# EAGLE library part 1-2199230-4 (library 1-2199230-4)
M.2 NGFF, M.2 Connectors, Height 4.2 mm [.165 in], Keying Code M, Gold, Board-to-Board, 67 Position, .02 in [.5 mm] Centerline, Printed Circuit Board Source: Datasheet
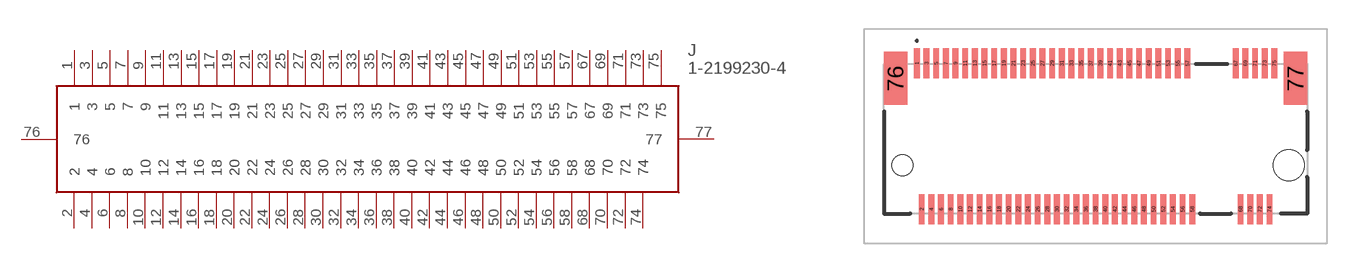
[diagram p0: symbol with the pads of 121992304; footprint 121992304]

Designator prefix J

## 1-2199230-4 (Arrow_Part_Number: 1-2199230-4; Arrow_Price-Stock: https://www.arrow.com/en/products/1-2199230-4/te-connectivity?region=nac; Description: M.2 NGFF, M.2 Connectors, Height 4.2 mm [.165 in], Keying Code M, Gold, Board-to-Board, 67 Position, .02 in [.5 mm] Centerline, Printed Circuit Board; Height: mm; Manufacturer_Name: TE Connectivity; Manufacturer_Part_Number: 1-2199230-4; Mouser_Part_Number: 571-1-2199230-4; Mouser_Price-Stock: https://www.mouser.co.uk/ProductDetail/TE-Connectivity/1-2199230-4?qs=gAfoL%252BRo%2FrJHWNmRjPOT7g%3D%3D)  [121992304]
1  1
2  2
3  3
4  4
5  5
6  6
7  7
8  8
9  9
10  10
11  11
12  12
13  13
14  14
15  15
16  16
17  17
18  18
19  19
20  20
21  21
22  22
23  23
24  24
25  25
26  26
27  27
28  28
29  29
30  30
31  31
32  32
33  33
34  34
35  35
36  36
37  37
38  38
39  39
40  40
41  41
42  42
43  43
44  44
45  45
46  46
47  47
48  48
49  49
50  50
51  51
52  52
53  53
54  54
55  55
56  56
57  57
58  58
67  67
68  68
69  69
70  70
71  71
72  72
73  73
74  74
75  75
76  76
77  77

## Footprint 121992304 (pad centres in mm)
1-2199230-4-3
smd 0.3 x 1.55: 1 -9.25,3.9; 2 -9,-3.65; 3 -8.75,3.9; 4 -8.5,-3.65; 5 -8.25,3.9; 6 -8,-3.65; 7 -7.75,3.9; 8 -7.5,-3.65; 9 -7.25,3.9; 10 -7,-3.65; 11 -6.75,3.9; 12 -6.5,-3.65; 13 -6.25,3.9; 14 -6,-3.65; 15 -5.75,3.9; 16 -5.5,-3.65; 17 -5.25,3.9; 18 -5,-3.65; 19 -4.75,3.9; 20 -4.5,-3.65; 21 -4.25,3.9; 22 -4,-3.65; 23 -3.75,3.9; 24 -3.5,-3.65; 25 -3.25,3.9; 26 -3,-3.65; 27 -2.75,3.9; 28 -2.5,-3.65; 29 -2.25,3.9; 30 -2,-3.65; 31 -1.75,3.9; 32 -1.5,-3.65; 33 -1.25,3.9; 34 -1,-3.65; 35 -0.75,3.9; 36 -0.5,-3.65; 37 -0.25,3.9; 38 0,-3.65; 39 0.25,3.9; 40 0.5,-3.65; 41 0.75,3.9; 42 1,-3.65; 43 1.25,3.9; 44 1.5,-3.65; 45 1.75,3.9; 46 2,-3.65; 47 2.25,3.9; 48 2.5,-3.65; 49 2.75,3.9; 50 3,-3.65; 51 3.25,3.9; 52 3.5,-3.65; 53 3.75,3.9; 54 4,-3.65; 55 4.25,3.9; 56 4.5,-3.65; 57 4.75,3.9; 58 5,-3.65; 67 7.25,3.9; 68 7.5,-3.65; 69 7.75,3.9; 70 8,-3.65; 71 8.25,3.9; 72 8.5,-3.65; 73 8.75,3.9; 74 9,-3.65; 75 9.25,3.9
smd 1.2 x 2.75: 76 -10.35,3.125; 77 10.35,3.125
hole 1.1 at -10,-1.375
hole 1.6 at 10,-1.375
